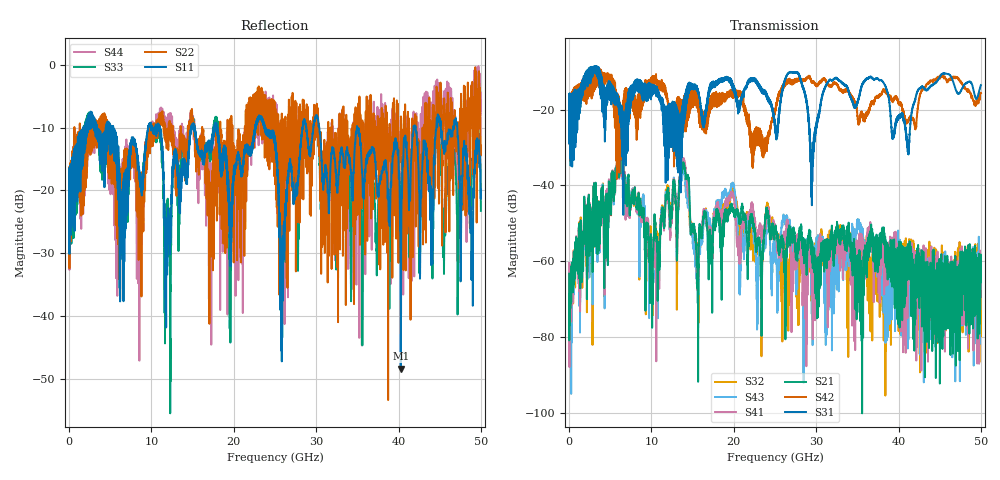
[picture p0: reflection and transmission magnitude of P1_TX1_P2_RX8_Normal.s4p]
!Keysight Technologies,N5225B,MY57041031,A.13.20.10
!Date: Friday, May 31, 2019 11:40:05
!Correction: S11(Full 4 Port(1,2,3,4))
!S12(Full 4 Port(1,2,3,4))
!S13(Full 4 Port(1,2,3,4))
!S14(Full 4 Port(1,2,3,4))
!S21(Full 4 Port(1,2,3,4))
!S22(Full 4 Port(1,2,3,4))
!S23(Full 4 Port(1,2,3,4))
!S24(Full 4 Port(1,2,3,4))
!S31(Full 4 Port(1,2,3,4))
!S32(Full 4 Port(1,2,3,4))
!S33(Full 4 Port(1,2,3,4))
!S34(Full 4 Port(1,2,3,4))
!S41(Full 4 Port(1,2,3,4))
!S42(Full 4 Port(1,2,3,4))
!S43(Full 4 Port(1,2,3,4))
!S44(Full 4 Port(1,2,3,4))
!S4P File: Measurements: <S11,S12,S13,S14>,
!<S21,S22,S23,S24>,
!<S31,S32,S33,S34>,
!<S41,S42,S43,S44>:
# Hz S  dB  R 50.0
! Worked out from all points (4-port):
!   5000 points, 10 MHz to 50 GHz, reference 50 ohm
!   strongest paths, dB at 10 MHz, 12.51 GHz, 25.01 GHz, 37.51 GHz, 50 GHz:
!     S31: -19.4, -29.2, -24.6, -11.8, -13.5
!     S42: -19.5, -21.6, -19.9, -16.5, -15.7
!     S21: -63.3, -46.8, -51.6, -62.1, -63.3
!     S41: -60.4, -48.3, -50.6, -58.0, -62.4
!     S43: -64.1, -45.8, -52.8, -57.2, -61.3
!     S32: -66.4, -44.9, -51.7, -59.4, -63.2
!   lowest |S11| = -48.4 dB at 40.27 GHz (marker M1), VSWR 1.01, Z = 49.7 + j0.165 ohm
!   |S11| at or under -10 dB: 18.01 GHz to 22.61 GHz (4.596 GHz wide, 22.6 % of centre); 30.38 GHz to 34.94 GHz (4.561 GHz wide, 14 % of centre); 34.98 GHz to 41.81 GHz (6.836 GHz wide, 17.8 % of centre)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
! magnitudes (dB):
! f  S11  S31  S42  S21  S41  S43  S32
! 10 MHz  -19.9  -19.4  -19.5  -63.3  -60.4  -64.1  -66.4
! 10.75 GHz  -9.6  -15.6  -12.6  -70.5  -63.3  -72.0  -63.6
! 13.89 GHz  -16.7  -17.5  -20.5  -34.0  -33.0  -34.5  -34.9
! 15.52 GHz  -12.9  -13.7  -16.8  -59.1  -66.0  -64.1  -55.8
! 19.84 GHz  -21.0  -13.1  -16.0  -46.2  -42.4  -39.5  -41.4
! 40.27 GHz  -48.4  -21.4  -18.3  -62.4  -59.5  -61.5  -55.9
! 50 GHz  -19.9  -13.5  -15.7  -63.3  -62.4  -61.3  -63.2
